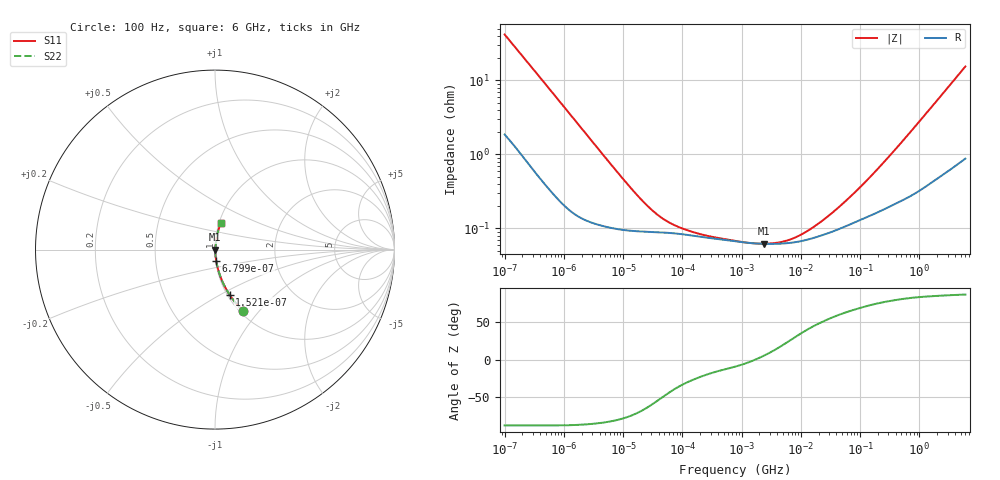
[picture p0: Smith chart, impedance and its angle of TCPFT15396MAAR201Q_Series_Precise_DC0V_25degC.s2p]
! TCPFT15396MAAR201Q Polymer Tantalum Capacitor Sparameter Model
! Model Generated by Samsung Electro-Mechanics
! Samsung Sparameter Version 5.0
! Date : Oct-21-2025
! Products : Polymer Tantalum Capacitor
! Characteristics :
!  Nominal Capacitance = 39uF
!  Capacitance Tolerance = +/-20%
!  ESR = 200 mohm max at 100kHz
!  Rated Voltage = 15Vdc
!  Size = 1206(unit:inch), 3216(unit:mm)
!  Length = 3.20+/-0.20mm
!  Width = 1.60+/-0.20mm
!  Thickness = 1.10+/-0.10mm
!  Lineup = Conductive Polymer Type
!  Feature = PFT
!  Measurement Temperature : 25degC.
!  DC bias Value = 0V
!  Frequency : 100Hz ~ 6GHz
! External Node Assignments :
!  1  o---||---o  2
# MHz S RI R 50.0
! Freq.  Real(S11)  Im(S11)  Real(S12)  Im(S12)  Real(S21)  Im(S21)  Real(S22)  Im(S22)
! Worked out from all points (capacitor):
!   300 points, 100 Hz to 6 GHz, reference 50 ohm
!   read as one part in series: C = 37.9 uF near 106.2 Hz
!   lowest |Z| = 62.2 mohm at 2.346 MHz (marker M1)
!   series resonance near 1.694 MHz, so ESL is about 230 pH
!   S11 on the Smith chart (normalised r, x): 100 Hz: 1.04, -0.83; 152.1 Hz: 1.02, -0.55; 679.9 Hz: 1.01, -0.13; 6 GHz: 1.02, +0.31
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0.0001  0.1587 -0.3437  0.8413 0.3437  0.8413 0.3437  0.1587 -0.3437
0.0001520888  0.0813 -0.2517  0.9187 0.2517  0.9187 0.2517  0.0813 -0.2517
0.0003120785  0.0243 -0.1338  0.9757 0.1338  0.9757 0.1338  0.0243 -0.1338
0.0006798988  0.00694 -0.0639  0.9931 0.0639  0.9931 0.0639  0.00694 -0.0639
0.001998454  0.00186 -0.0222  0.9981 0.0222  0.9981 0.0222  0.00186 -0.0222
0.01531674  0.000929 -0.00299  0.9991 0.00299  0.9991 0.00299  0.000929 -0.00299
0.02625979  0.000902 -0.00177  0.9991 0.00177  0.9991 0.00177  0.000902 -0.00177
0.03993819  0.000887 -0.00119  0.9991 0.00119  0.9991 0.00119  0.000887 -0.00119
0.06847205  0.000861 -0.000741  0.9991 0.000741  0.9991 0.000741  0.000861 -0.000741
0.1323324  0.000809 -0.000443  0.9992 0.000443  0.9992 0.000443  0.000809 -0.000443
0.2715393  0.000746 -0.00026  0.9993 0.00026  0.9993 0.00026  0.000746 -0.00026
0.7981464  0.000667 -0.000106  0.9993 0.000106  0.9993 0.000106  0.000667 -0.000106
2.346024  0.000619 5.49e-05  0.9994 -5.49e-05  0.9994 -5.49e-05  0.000619 5.49e-05
6.117227  0.000633 0.000282  0.9994 -0.000282  0.9994 -0.000282  0.000633 0.000282
9.877924  0.000671 0.000464  0.9993 -0.000464  0.9993 -0.000464  0.000671 0.000464
15.95059  0.000738 0.000716  0.9993 -0.000716  0.9993 -0.000716  0.000738 0.000716
30.82687  0.000879 0.00124  0.9991 -0.00124  0.9991 -0.00124  0.000879 0.00124
63.25518  0.00111 0.00227  0.9989 -0.00227  0.9989 -0.00227  0.00111 0.00227
137.8087  0.00146 0.00442  0.9985 -0.00442  0.9985 -0.00442  0.00146 0.00442
318.7652  0.00206 0.00941  0.9979 -0.00941  0.9979 -0.00941  0.00206 0.00941
1922.593  0.00717 0.0508  0.9928 -0.0508  0.9928 -0.0508  0.00717 0.0508
6000  0.0313 0.1478  0.9687 -0.1478  0.9687 -0.1478  0.0313 0.1478
